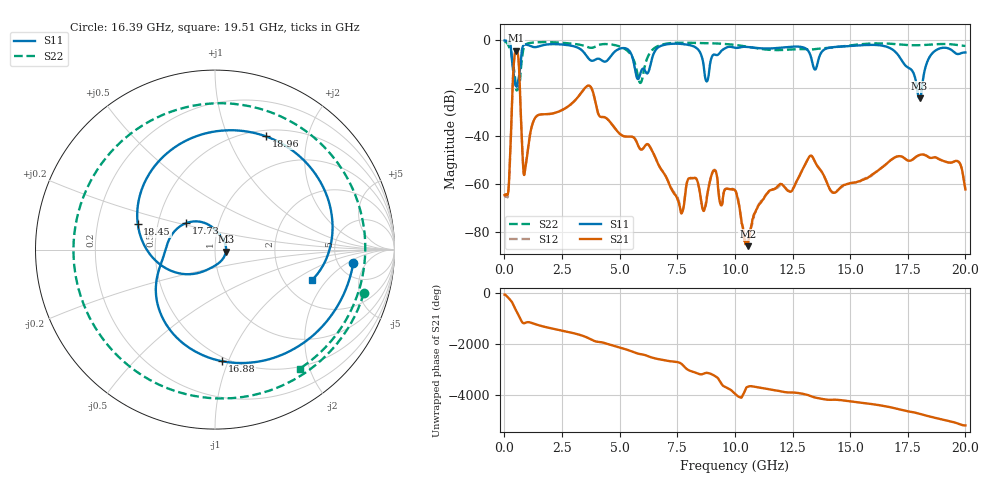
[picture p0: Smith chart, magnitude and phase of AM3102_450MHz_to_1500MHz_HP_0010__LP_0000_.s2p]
!Agilent Technologies,E8364B,MY43040894,A.07.50.67
!Agilent E8364B: A.07.50.67
!Date: Thursday, January 11, 2018 05:23:34
!Correction: S11(Full 2 Port(1,2))
!S21(Full 2 Port(1,2))
!S12(Full 2 Port(1,2))
!S22(Full 2 Port(1,2))
!S2P File: Measurements: S11, S21, S12, S22:
# Hz S  dB  R 50
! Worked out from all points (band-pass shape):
!   1601 points, 10 MHz to 20 GHz, reference 50 ohm
!   highest |S21| = -4.31 dB at 509.8 MHz (marker M1); lowest = -85.7 dB at 10.55 GHz (marker M2)
!   |S21| within 3 dB of the highest: 431.8 MHz to 605.9 MHz (174.1 MHz wide, 33.6 % of centre)
!   lowest |S11| = -24.2 dB at 18.01 GHz (marker M3), VSWR 1.13, Z = 56.5 - j1.24 ohm
!   |S11| at or under -10 dB: 346 MHz to 702.1 MHz (356.1 MHz wide, 68 % of centre); 5.626 GHz to 6.343 GHz (717 MHz wide, 12 % of centre); 17.35 GHz to 18.31 GHz (952.2 MHz wide, 5.34 % of centre)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
!   |S22| runs from -20.9 to -0.4 dB; largest |S21 - S12| = 0.0025
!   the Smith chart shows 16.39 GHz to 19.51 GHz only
!   S11 on the Smith chart (normalised r, x): 16.39 GHz: 6.89, -2.56; 16.88 GHz: 0.47, -0.95; 17.73 GHz: 0.70, +0.22; 18.45 GHz: 0.38, +0.14; 18.96 GHz: 0.57, +1.39; 19.51 GHz: 2.86, -1.41
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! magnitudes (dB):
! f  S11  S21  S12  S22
! 10 MHz  -0.1  -64.4  -64.1  -0.4
! 172.4 MHz  -0.6  -62.8  -63.5  -2.2
! 509.8 MHz  -18.5  -4.3  -4.3  -20.3
! 884.6 MHz  -1.8  -54.7  -54.6  -2.1
! 1.359 GHz  -2.8  -32.0  -32.0  -0.8
! 3.346 GHz  -4.0  -21.7  -21.7  -2.0
! 5.895 GHz  -14.0  -45.3  -45.3  -17.8
! 6.682 GHz  -2.9  -51.7  -51.6  -2.3
! 7.681 GHz  -1.5  -72.1  -71.1  -1.0
! 8.781 GHz  -17.1  -65.7  -65.0  -1.2
! 10.01 GHz  -3.1  -62.4  -62.5  -1.9
! 10.55 GHz  -2.8  -85.7  -84.1  -2.7
! 13.34 GHz  -8.4  -48.2  -48.2  -3.8
! 16.39 GHz  -2.2  -52.9  -52.9  -1.3
! 16.68 GHz  -3.0  -50.6  -50.5  -1.4
! 16.88 GHz  -4.1  -49.1  -49.1  -1.5
! 17.73 GHz  -13.2  -49.5  -49.6  -2.1
! 18.01 GHz  -24.2  -47.7  -47.7  -2.0
! 18.45 GHz  -6.9  -48.9  -48.9  -1.8
! 18.96 GHz  -3.2  -49.9  -50.0  -1.5
! 19.51 GHz  -4.9  -50.5  -50.5  -1.8
! 20 GHz  -5.1  -62.1  -61.6  -2.4
